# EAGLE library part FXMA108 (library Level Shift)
FXMA108 level shifter.
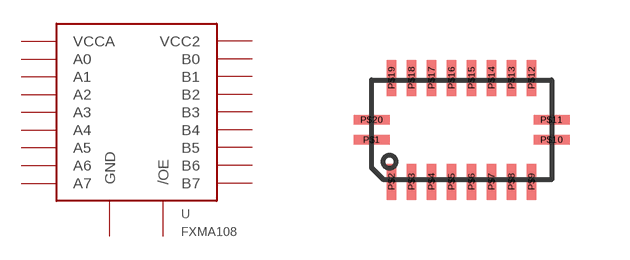
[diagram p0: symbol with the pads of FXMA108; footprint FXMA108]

Designator prefix U

## FXMA108  [FXMA108]
P$1  VCCA
P$2  A0
P$3  A1
P$4  A2
P$5  A3
P$6  A4
P$7  A5
P$8  A6
P$9  A7
P$10  GND
P$11  /OE
P$12  B0
P$13  B1
P$14  B2
P$15  B3
P$16  B4
P$17  B5
P$18  B6
P$19  B7
P$20  VCC2

## Footprint FXMA108 (pad centres in mm)
FXMA108
smd 0.9 x 0.24: P$1 -2.25,-0.25; P$10 2.25,-0.25; P$11 2.25,0.25; P$20 -2.25,0.25
smd 0.24 x 0.9: P$2 -1.75,-1.3; P$3 -1.25,-1.3; P$4 -0.75,-1.3; P$5 -0.25,-1.3; P$6 0.25,-1.3; P$7 0.75,-1.3; P$8 1.25,-1.3; P$9 1.75,-1.3; P$12 1.75,1.3; P$13 1.25,1.3; P$14 0.75,1.3; P$15 0.25,1.3; P$16 -0.25,1.3; P$17 -0.75,1.3; P$18 -1.25,1.3; P$19 -1.75,1.3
